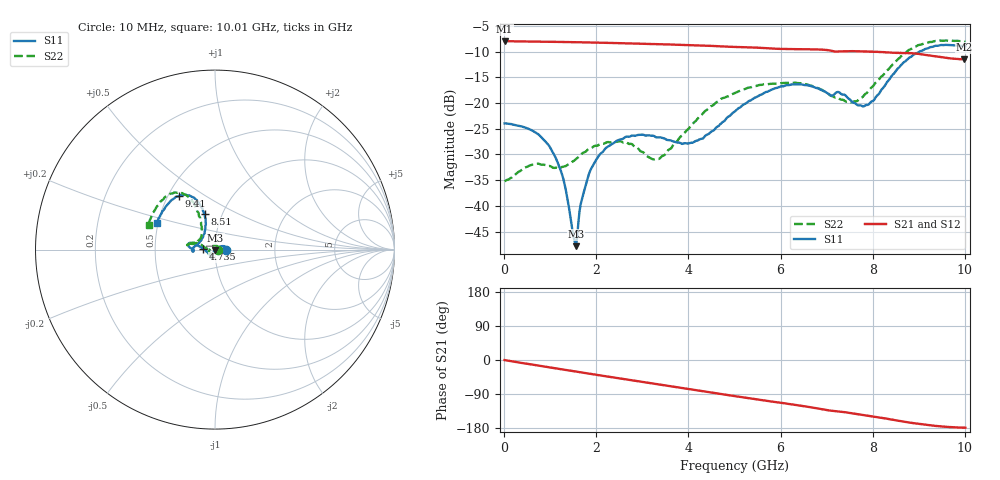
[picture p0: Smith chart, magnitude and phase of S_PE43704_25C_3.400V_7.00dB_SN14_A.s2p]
! Device ID: PE43704
! Dir: z:\PE43704\PE43704_Char_1_20130516\PE43704\AMB\3p400V\7p00dB
! Serial: 14
! Insertion: A
! Impedance: 50 ohm
! Temp: Amb
! VDD: 3.400V
! Attenuation Step: 7.00dB
! IDD: 1.140365e-01mA
#  Hz  S  RI  R  50
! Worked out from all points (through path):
!   401 points, 10 MHz to 10.01 GHz, reference 50 ohm
!   highest |S21| = -7.99 dB at 10 MHz (marker M1); lowest = -11.5 dB at 9.985 GHz (marker M2)
!   group delay of S21, straight-line fit = 51 ps
!   lowest |S11| = -47.8 dB at 1.56 GHz (marker M3), VSWR 1.01, Z = 50.2 - j0.372 ohm
!   |S11| at or under -10 dB: start of sweep to 9.018 GHz
!   |S22| runs from -35.2 to -7.9 dB; largest |S21 - S12| = 0.0026
!   S11 on the Smith chart (normalised r, x): 10 MHz: 1.14, +0.00; 4.735 GHz: 0.88, +0.01; 8.51 GHz: 0.83, +0.34; 9.41 GHz: 0.57, +0.39; 10.01 GHz: 0.49, +0.17
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1e7  0.0633 0.000231  0.3985 -0.00155  0.3988 -0.00143  0.0173 0.00042
6.1e8  0.0504 0.0195  0.3861 -0.0832  0.3861 -0.083  0.00843 0.0237
9.85e8  0.0329 0.0186  0.3707 -0.1305  0.3706 -0.1304  -0.00558 0.0238
1.26e9  0.0176 0.00951  0.3553 -0.1642  0.3554 -0.164  -0.0182 0.0156
1.51e9  0.00451 -0.00198  0.3387 -0.1924  0.3388 -0.1922  -0.027 0.00437
1.56e9  0.00167 -0.0037  0.3353 -0.1979  0.3353 -0.1978  -0.0285 0.00185
1.685e9  -0.00383 -0.0108  0.3258 -0.2116  0.3259 -0.2114  -0.0319 -0.00425
1.885e9  -0.0111 -0.02  0.3095 -0.2319  0.3097 -0.2316  -0.0338 -0.0132
2.235e9  -0.0176 -0.0329  0.2782 -0.2643  0.2783 -0.2641  -0.0352 -0.0223
3.36e9  -0.0213 -0.0412  0.1586 -0.3367  0.1591 -0.3365  -0.027 -0.00948
4.06e9  -0.0348 -0.0219  0.0763 -0.356  0.0767 -0.3559  -0.0586 0.0135
4.735e9  -0.065 0.00358  -0.00324 -0.3542  -0.00286 -0.3545  -0.1051 0.0365
5.01e9  -0.0816 0.015  -0.033 -0.3487  -0.0327 -0.349  -0.1209 0.0323
5.96e9  -0.1371 0.038  -0.1267 -0.3109  -0.1256 -0.3112  -0.1521 0.0303
6.685e9  -0.1443 0.0147  -0.1923 -0.2707  -0.1925 -0.2701  -0.1427 0.0322
7.585e9  -0.095 0.0322  -0.2487 -0.1992  -0.2484 -0.199  -0.0792 0.0664
7.935e9  -0.0652 0.0752  -0.2669 -0.1684  -0.2672 -0.1691  -0.0741 0.114
8.36e9  -0.0523 0.1614  -0.2826 -0.1254  -0.2821 -0.1266  -0.0906 0.1979
8.51e9  -0.0575 0.198  -0.2869 -0.108  -0.286 -0.1094  -0.1048 0.234
9.41e9  -0.2024 0.2968  -0.2806 -0.0271  -0.2802 -0.0264  -0.2639 0.3003
9.985e9  -0.3182 0.1586  -0.2646 -0.00661  -0.2653 -0.00592  -0.3664 0.1466
1.001e10  -0.3238 0.1483  -0.2656 -0.00653  -0.267 -0.00624  -0.3702 0.1382
